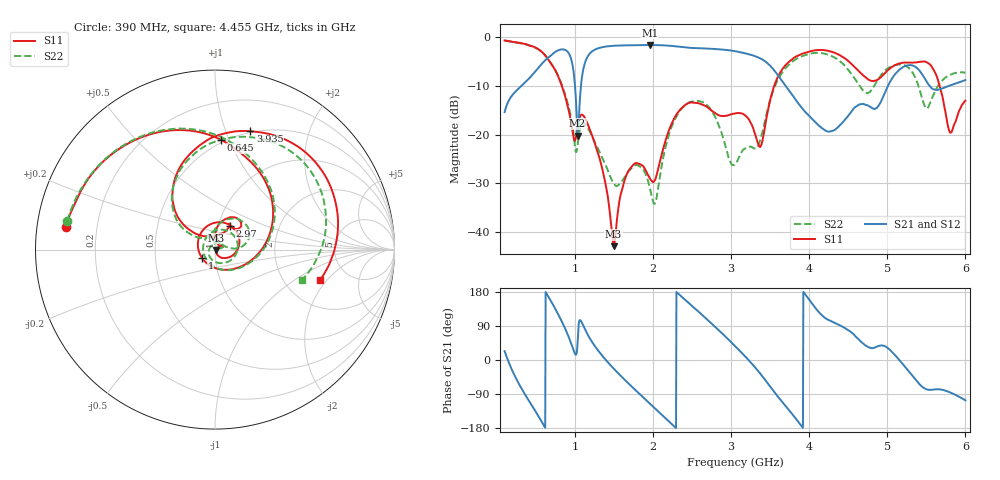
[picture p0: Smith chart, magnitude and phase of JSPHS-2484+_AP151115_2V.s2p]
!Mini-Circuits Laboratory
!S-Parameters
!Run/Lot/Date Code:MF33450/NA/1551
!Fixture/SN/Due: 90-4-20-21/70546/03/17/16
!Connection:PORT<IN> - pin<1>; PORT<OUT> - pin<7>;PORT<BIAS> - pin<4>;
!Tested With:PORT EXTENTION
!Network Analyzer:AG E5071C/74883/05/12/16
!Created: 01-07-2016 at 14:09:11
!MODEL: JSPHS-2484+
!S/N: V=2V
# MHZ S DB R 50
!Frequency  S11 dB  S11 DEG  S21 dB  S21 DEG  S12 dB  S12 DEG  S22 dB  S22 DEG
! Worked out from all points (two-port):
!   1181 points, 100 MHz to 6 GHz, reference 50 ohm
!   highest |S21| = -1.59 dB at 1.96 GHz (marker M1); lowest = -20.2 dB at 1.035 GHz (marker M2)
!   |S21| within 3 dB of the highest: 628.8 MHz to 954 MHz (325.2 MHz wide, 41.1 % of centre); 1.144 GHz to 3.403 GHz (2.259 GHz wide, 99.4 % of centre)
!   lowest |S11| = -43.0 dB at 1.495 GHz (marker M3), VSWR 1.01, Z = 50.7 - j0.185 ohm
!   |S11| at or under -10 dB: 832.5 MHz to 3.551 GHz (2.719 GHz wide, 124 % of centre); 5.67 GHz to end of sweep
!   |S22| runs from -34.3 to -0.7 dB; largest |S21 - S12| = 0.0034
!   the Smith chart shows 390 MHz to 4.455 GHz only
!   S11 on the Smith chart (normalised r, x): 390 MHz: 0.09, +0.07; 645 MHz: 0.48, +0.94; 1 GHz: 0.86, -0.08; 2.97 GHz: 1.14, +0.31; 3.935 GHz: 0.49, +1.22; 4.455 GHz: 3.13, -1.69
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100  -0.65 -66.3  -15.40 23.3  -15.39 23.3  -0.65 -66.4
390  -1.50 171.4  -8.85 -100.8  -8.84 -100.8  -1.53 169.0
645  -4.26 86.8  -4.37 172.2  -4.36 172.2  -4.21 84.1
850  -10.84 7.9  -2.49 94.1  -2.49 94.1  -10.54 8.2
1000  -21.26 -148.0  -9.72 16.5  -9.71 16.5  -22.30 -121.4
1035  -18.36 131.1  -20.20 49.3  -20.20 49.3  -22.08 134.8
1085  -15.93 61.7  -8.92 100.3  -8.91 100.3  -17.90 51.3
1495  -42.97 -14.9  -1.74 -22.3  -1.74 -22.3  -30.00 171.9
1690  -27.36 34.1  -1.64 -62.7  -1.64 -62.7  -27.51 61.8
1960  -29.03 29.2  -1.59 -115.2  -1.59 -115.2  -31.05 14.8
2070  -26.82 78.9  -1.61 -136.4  -1.61 -136.4  -30.59 91.1
2470  -13.44 56.5  -2.15 148.1  -2.15 148.1  -13.33 50.8
2970  -16.01 57.6  -2.66 53.2  -2.66 53.2  -24.83 19.1
3050  -15.63 60.5  -2.85 36.9  -2.85 36.8  -26.12 58.4
3470  -15.16 142.2  -5.39 -61.8  -5.39 -61.9  -14.70 147.6
3935  -3.24 73.4  -15.10 177.1  -15.10 177.4  -3.73 74.7
4035  -2.79 58.6  -16.77 149.3  -16.75 149.2  -3.29 58.7
4455  -4.31 -16.2  -17.01 84.7  -17.08 85.4  -5.84 -19.3
5020  -6.59 139.8  -9.62 29.3  -9.62 29.1  -6.24 107.8
5500  -5.10 22.4  -9.01 -77.2  -9.07 -77.0  -14.64 58.9
5805  -19.61 3.3  -9.90 -85.5  -9.86 -85.5  -7.73 72.4
6000  -13.04 29.8  -8.80 -106.6  -8.78 -106.6  -7.30 56.5
